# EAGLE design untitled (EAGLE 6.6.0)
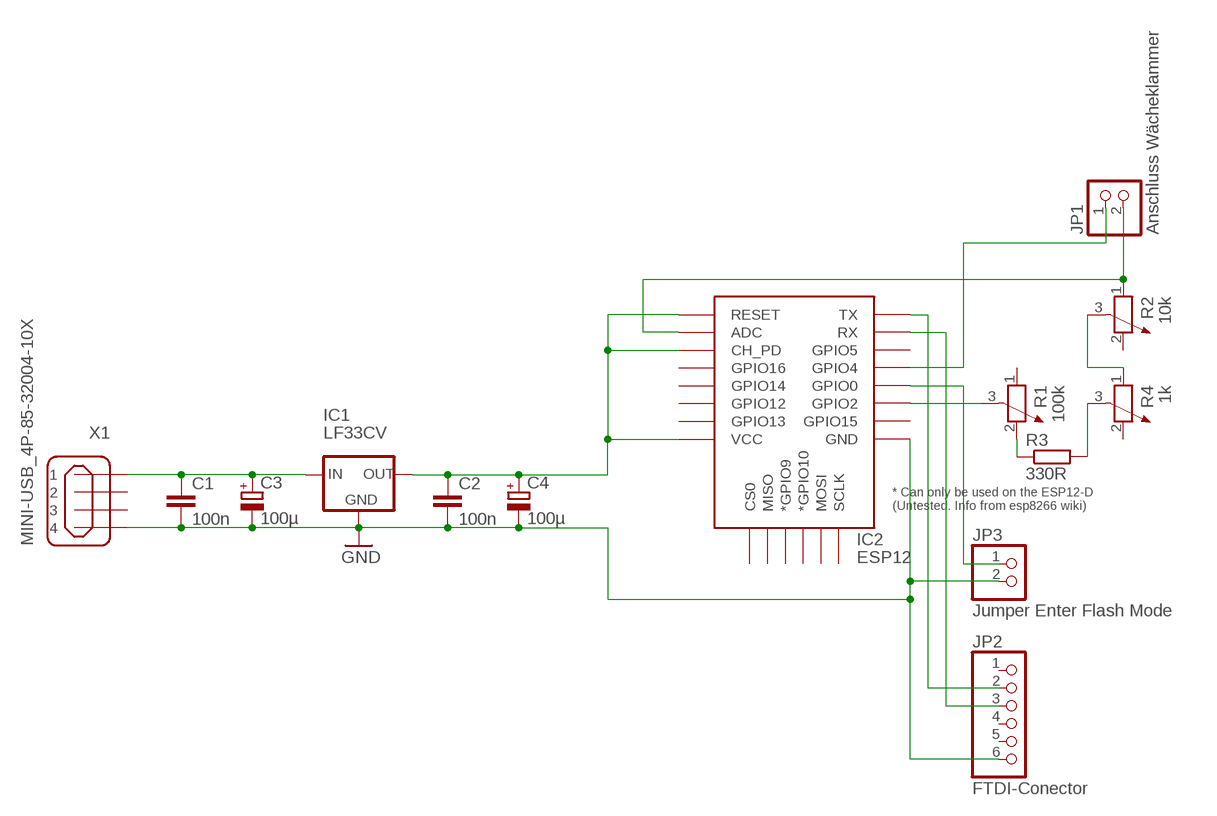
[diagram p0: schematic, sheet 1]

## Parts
C1  100n  C-EU025-030X050  [C025-030X050]
C2  100n  C-EU025-030X050  [C025-030X050]
C3  100µ  CPOL-EUE2.5-7  [E2,5-7]
C4  100µ  CPOL-EUE2.5-7  [E2,5-7]
IC1  LF33CV  78XXS  [78XXS]
IC2  ESP12  ESP12ESMD  [ESP12E-SMD]
JP1  Anschluss Wächeklammer  PINHD-1X2  [1X02]
JP2  FTDI-Conector  PINHD-1X6  [1X06]
JP3  Jumper Enter Flash Mode  PINHD-1X2  [1X02]
R1  100k  POTENTIOMETER_PT-10  [PT-10]
R2  10k  POTENTIOMETER_PT-10  [PT-10]
R3  330R  R-EU_0207/10  [0207/10]
R4  1k  POTENTIOMETER_PT-10  [PT-10]
X1  MINI-USB_4P-85-32004-10X  [85-32004-10X]

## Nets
GND [GND]: C1.2 C2.2 C3.- C4.- IC1.GND IC2.GND JP2.6 JP3.2 X1.4
N$1 [VCC]: C1.1 C3.+ IC1.IN X1.1
N$2 [VCC]: C2.1 C4.+ IC1.OUT IC2.CH_PD IC2.RESET IC2.VCC
N$3: IC2.GPIO2 R1.3
N$4: R2.3 R4.1
N$5: IC2.GPIO4 JP1.1
N$6: IC2.ADC JP1.2 R2.1
N$7: IC2.GPIO0 JP3.1
N$9: IC2.TXD0(TX) JP2.2
N$10: IC2.RXD0(RX) JP2.3
N$11: R1.2 R3.1
N$12: R3.2 R4.3
Unconnected: IC2.CS0 IC2.GPIO5 IC2.GPIO9(*GPIO9) IC2.GPIO10(*GPIO10) IC2.GPIO12 IC2.GPIO13 IC2.GPIO14 IC2.GPIO15 IC2.GPIO16 IC2.MISO IC2.MOSI IC2.SCLK JP2.1 JP2.4 JP2.5 R1.1 R2.2 R4.2 X1.2 X1.3

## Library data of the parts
C1 C2 = rcl:C-EU: CAPACITOR, European symbol
C3 C4 = rcl:CPOL-EU: POLARIZED CAPACITOR, European symbol
IC1 = v-reg:78XXS: VOLTAGE REGULATOR
IC2 = esp8266modules:ESP12E: ESP12E Module
JP1 JP3 = pinhead:PINHD-1X2: PIN HEADER
JP2 = pinhead:PINHD-1X6: PIN HEADER
R1 R2 R4 = rcl:POTENTIOMETER_: Potentiometer
R3 = rcl:R-EU_: RESISTOR, European symbol
X1 = con-cypressindustries:MINI-USB_4P-: MINI USB 4 Pol. Source: www.cypressindustries.com; OC_FARNELL: unknown; OC_NEWARK: unknown

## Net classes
0 default: width 0.051 mm, drill 0.051 mm, clearance 0.127 mm
1 VCC: width 0.203 mm, drill 0.152 mm, clearance 0.127 mm
2 GND: width 0.203 mm, drill 0.152 mm, clearance 0.127 mm

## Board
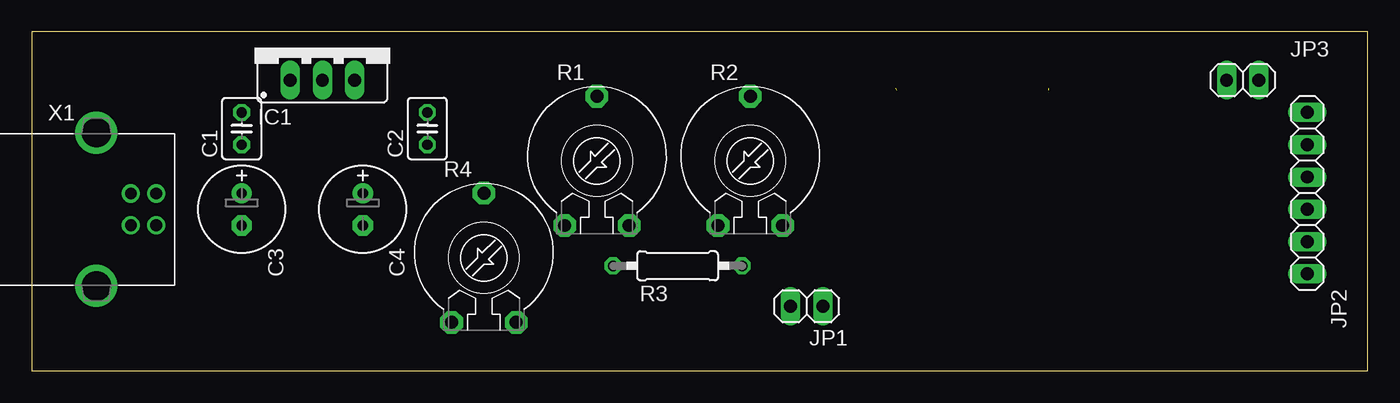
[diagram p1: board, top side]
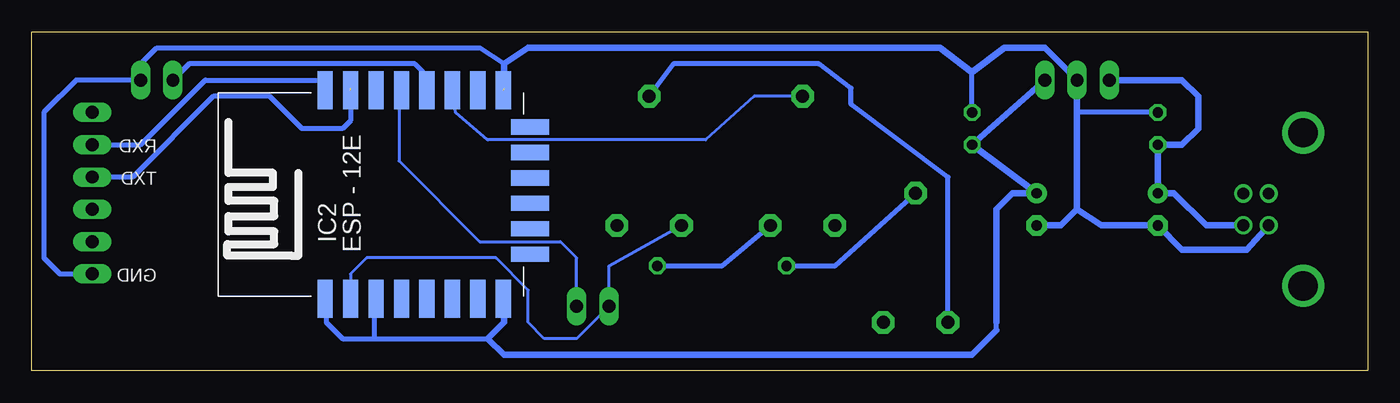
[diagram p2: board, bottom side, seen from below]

Size 105.08 x 26.66 mm. Coordinates in mm from the lower left corner, seen from the top.
Outline: 0,0 105.08,0 105.08,26.66 0,26.66 0,0
Copper layers (1*16): Top 0.035mm / dielectric 1.5mm / Bottom 0.035mm
Design rules "default": minimum track width 10mil, minimum drill 24mil, track to track 8mil, track to pad 8mil, pad to pad 8mil, via to via 8mil, smd to smd 8mil, copper to edge 40mil, drill to drill 8mil, minimum pad ring 10mil, minimum via ring 8mil, stop-mask expansion 4mil, vias tented up to drill 0mil, thermal gap 10mil

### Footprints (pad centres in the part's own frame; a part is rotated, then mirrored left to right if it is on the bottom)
C025-030X050 = drill 0.813 octagon: 1 -1.27,0; 2 1.27,0
E2,5-7 = drill 0.813 pad 1.6: + -1.27,0 | drill 0.813 pad 1.6 octagon: - 1.27,0
78XXS = drill 1.016 long: GND 0,-2.54; IN -2.54,-2.54; OUT 2.54,-2.54
ESP12E-SMD = smd 3 x 1.2: ADC -8.3,3.8; CH_PD -8.3,1.8; GND 8.1,-8.2; GPIO0 8.1,-2.2; GPIO2 8.1,-4.2; GPIO4 8.1,-0.2; GPIO5 8.1,1.8; GPIO12 -8.3,-4.2; GPIO13 -8.3,-6.2; GPIO14 -8.3,-2.2; GPIO15 8.1,-6.2; GPIO16 -8.3,-0.2; RESET -8.3,5.8; RXD0 8.1,3.8; TXD0 8.1,5.8; VCC -8.3,-8.2 | smd 1.2 x 3: CS0 -4.8,-10.3; GPIO9 -0.8,-10.3; GPIO10 1.2,-10.3; MISO -2.8,-10.3; MOSI 3.2,-10.3; SCLK 5.2,-10.3
1X02 = drill 1.016 long: 1 -1.27,0; 2 1.27,0
1X06 = drill 1.016 long: 1 -6.35,0; 2 -3.81,0; 3 -1.27,0; 4 1.27,0; 5 3.81,0; 6 6.35,0
PT-10 = drill 1.016 pad 1.778 octagon: 1 -2.54,-5.08; 2 2.54,-5.08; 3 0,5.08
0207/10 = drill 0.813 octagon: 1 -5.08,0; 2 5.08,0
85-32004-10X = drill 0.92 pad 1.27: 1 4.71,-1.25; 2 4.71,1.25; 3 2.71,1.25; 4 2.71,-1.25 | drill 2.3 pad 3: M1 0,6.02; M2 0,-6.02

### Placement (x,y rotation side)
C1  16.51,19.05 90 top
C2  31.11,19.05 90 top
C3  16.51,12.7 270 top
C4  26.04,12.7 270 top
IC1  22.86,25.4 0 top
IC2  76.2,13.97 90 bottom
JP1  60.96,5.08 180 top
JP2  100.33,13.97 270 top
JP3  95.25,22.86 0 top
R1  44.45,16.51 0 top
R2  56.52,16.51 0 top
R3  50.8,8.26 180 top
R4  35.56,8.89 0 top
X1  5.08,12.7 0 top

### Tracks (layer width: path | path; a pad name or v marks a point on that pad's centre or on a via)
GND  (1 unrouted)
  Bottom 0.406: C1.2 22.86,20.32 | JP2.6 102.87,7.62 104.14,8.89 104.14,20.32 101.6,22.86 JP3.2 96.52,24.13 95.25,25.4 69.85,25.4 67.95,24.13 | C2.2 31.11,23.49
  Bottom 0.508: X1.4 9.53,9.52 14.61,9.52 C3.- 20.95,11.43 22.86,12.7 | 22.86,12.7 22.86,20.32 IC1.GND 24.13,24.13 25.4,25.4 28.57,25.4 31.11,23.49 33.66,25.4 66.04,25.4 67.95,24.13 67.95,22.23 | C4.- 24.13,11.43 22.86,12.7
N$1
  Bottom 0.508: X1.1 12.7,11.43 15.24,13.97 C3.+ C1.1 14.61,17.78 13.34,19.05 13.34,21.59 14.61,22.86 IC1.IN
N$2
  Bottom 0.254: 81.92,5.08 IC2.RESET | 78.11,5.08 IC2.CH_PD
  Bottom 0.406: 78.11,2.54 80.65,2.54 81.92,3.81 81.92,5.08 | 78.11,2.54 69.22,2.54 | 78.11,2.54 78.11,5.08 | 67.95,5.08 68,5.08 IC2.VCC 67.95,5.67 67.95,3.81 | 29.21,3.17 29.21,3.81
  Bottom 0.508: IC1.OUT C2.1 C4.+ 27.94,13.97 29.21,12.7 29.21,3.81 | 67.95,5.08 67.95,3.81 69.22,2.54 67.95,1.27 31.11,1.27 29.21,3.17
N$3
  Bottom 0.254: R1.3 48.26,21.59 52.07,18.16 69.22,18.16 71.76,20.32 IC2.GPIO2
N$4
  Bottom 0.406: R4.1 33.02,15.24 40.64,20.95 40.64,22.23 43.18,24.13 54.61,24.13 R2.3
N$5
  Bottom 0.254: 76.2,22.07 76.2,16.51 69.85,10.16 63.5,10.16 62.23,8.89 JP1.1
  Bottom 0.406: IC2.GPIO4 76.2,22.07
N$6
  Bottom 0.254: IC2.ADC 80.01,6.35 80.01,7.62 78.74,8.89 68.58,8.89 66.04,6.35 66.04,3.81 64.77,2.54 62.23,2.54 JP1.2 59.69,8.26 R2.1
N$7
  Bottom 0.406: IC2.GPIO0 73.66,22.07 73.66,22.86 74.93,24.13 92.71,24.13 JP3.1
N$8
  Bottom 0.406: 81.92,4.45 81.92,3.81
N$9
  Bottom 0.406: JP2.2 96.52,17.78 91.44,22.86 82,22.86 | 81.92,22.86 82,22.86 | 82,22.86 IC2.TXD0
N$10  (1 unrouted)
  Bottom 0.406: IC2.RXD0 | JP2.3 97.16,15.24 90.81,21.59 86.36,21.59 83.82,19.05 80.65,19.05 80.01,19.68 80.01,22.23
N$11
  Bottom 0.406: R3.1 50.8,8.26 R1.2
N$12
  Bottom 0.406: R3.2 41.91,8.26 R4.3

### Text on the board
bPlace: RXD | TXD | GND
